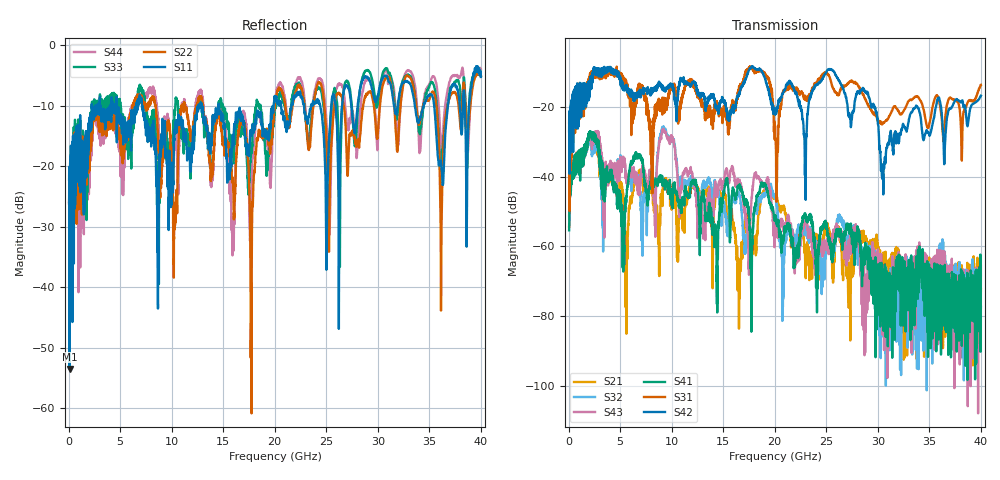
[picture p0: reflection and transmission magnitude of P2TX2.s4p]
!Agilent Technologies,N5245A,MY49151084,A.09.20.08
!Agilent N5245A: A.09.20.08
!Date: Thursday, March 01, 2012 14:14:03
!Correction: S11(Full 4 Port(1,2,3,4))
!S12(Full 4 Port(1,2,3,4))
!S13(Full 4 Port(1,2,3,4))
!S14(Full 4 Port(1,2,3,4))
!S21(Full 4 Port(1,2,3,4))
!S22(Full 4 Port(1,2,3,4))
!S23(Full 4 Port(1,2,3,4))
!S24(Full 4 Port(1,2,3,4))
!S31(Full 4 Port(1,2,3,4))
!S32(Full 4 Port(1,2,3,4))
!S33(Full 4 Port(1,2,3,4))
!S34(Full 4 Port(1,2,3,4))
!S41(Full 4 Port(1,2,3,4))
!S42(Full 4 Port(1,2,3,4))
!S43(Full 4 Port(1,2,3,4))
!S44(Full 4 Port(1,2,3,4))
!S4P File: Measurements: <S11,S12,S13,S14>,
!<S21,S22,S23,S24>,
!<S31,S32,S33,S34>,
!<S41,S42,S43,S44>:
# Hz S  dB  R 50
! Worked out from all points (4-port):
!   3996 points, 50 MHz to 40 GHz, reference 50 ohm
!   strongest paths, dB at 50 MHz, 10.04 GHz, 20.03 GHz, 30.02 GHz, 40 GHz:
!     S42: -27.0, -14.3, -21.8, -25.1, -16.8
!     S31: -24.7, -13.9, -25.5, -23.7, -13.7
!     S41: -55.4, -45.4, -51.2, -65.2, -77.4
!     S43: -54.3, -29.9, -56.4, -65.8, -65.6
!     S32: -51.3, -30.0, -45.9, -76.9, -68.3
!     S21: -54.4, -47.0, -46.1, -62.0, -72.3
!   lowest |S11| = -53.5 dB at 90 MHz (marker M1), VSWR 1.00, Z = 49.9 + j0.204 ohm
!   |S11| at or under -10 dB: start of sweep to 2.239 GHz; 7.123 GHz to 12.61 GHz (5.486 GHz wide, 55.6 % of centre); 14.57 GHz to 19.89 GHz (5.324 GHz wide, 30.9 % of centre)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
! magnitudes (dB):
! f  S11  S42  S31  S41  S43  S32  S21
! 50 MHz  -22.2  -27.0  -24.7  -55.4  -54.3  -51.3  -54.4
! 90 MHz  -53.5  -39.2  -49.9  -47.3  -47.3  -47.3  -47.3
! 9.24 GHz  -15.3  -14.8  -20.9  -41.8  -26.6  -25.9  -41.5
! 17.72 GHz  -14.7  -8.9  -9.1  -74.0  -48.0  -58.6  -61.1
! 20.78 GHz  -11.3  -16.0  -15.9  -59.0  -54.1  -72.2  -49.1
! 30.47 GHz  -5.5  -39.2  -24.6  -80.6  -85.4  -83.2  -64.9
! 40 GHz  -5.3  -16.8  -13.7  -77.4  -65.6  -68.3  -72.3
